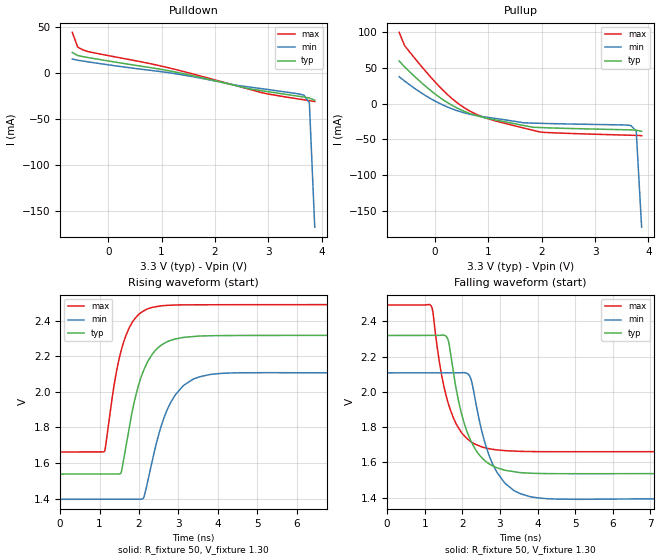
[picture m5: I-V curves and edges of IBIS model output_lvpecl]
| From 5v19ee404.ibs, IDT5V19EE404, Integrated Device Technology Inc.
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[Model]   output_lvpecl
Model_type   Output_ECL
Polarity   Non-Inverting
|   typ   min   max
C_comp   2pF   1.5pF   2.5pF
Vmeas = 1.95V
Rref = 50
Cref = 0
Vref = 1.3V
|   typ   min   max
[Voltage range]   3.3V   3.135V   3.465V
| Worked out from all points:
|   rising waveform, R_fixture 50, V_fixture 1.30: 20-80 % time 534ps typ, 606ps min, 451ps max; typ from 1.54 V to 2.32 V
|   falling waveform, R_fixture 50, V_fixture 1.30: 20-80 % time 574ps typ, 609ps min, 527ps max; typ from 2.32 V to 1.54 V
[Pulldown]
|Voltage   I (typ)   I (min)   I (max)
|Note, modeling breaks down at 250mA and above.  This is well beyond the functional   |
|operating range of the device.  Should this scenario occur, catastrophic failure and   |
|possible damage to the device and/or board is of higher concern than the I-V curve   |
|behavior.  The IBIS checker will flag currents in excess of 10A with warnings.  Lines   |
|with currents in excess of 0.35 A have been commented out.  The points still remain|
|available to the user if the user desires to use them.   |
|-3.30000e+00   3.30641e+01   2.49914e+01   4.38849e+01
|-3.19898e+00   3.16607e+01   2.38842e+01   4.20980e+01
|-3.09796e+00   3.02581e+01   2.27777e+01   4.03117e+01
|-2.99694e+00   2.88562e+01   2.16720e+01   3.85264e+01
|-2.89592e+00   2.74551e+01   2.05672e+01   3.67423e+01
|-2.79490e+00   2.60551e+01   1.94634e+01   3.49594e+01
|-2.69388e+00   2.46561e+01   1.83607e+01   3.31775e+01
|-2.59286e+00   2.32583e+01   1.72592e+01   3.13966e+01
|-2.49184e+00   2.18620e+01   1.61591e+01   2.96168e+01
|-2.39082e+00   2.04675e+01   1.50607e+01   2.78382e+01
|-2.28980e+00   1.90751e+01   1.39641e+01   2.60611e+01
|-2.18878e+00   1.76846e+01   1.28696e+01   2.42857e+01
|-2.08776e+00   1.62964e+01   1.17779e+01   2.25121e+01
|-1.98673e+00   1.49107e+01   1.06894e+01   2.07407e+01
|-1.88571e+00   1.35280e+01   9.60463e+00   1.89718e+01
|-1.78469e+00   1.21491e+01   8.52420e+00   1.72060e+01
|-1.68367e+00   1.07746e+01   7.44910e+00   1.54439e+01
|-1.58265e+00   9.40591e+00   6.38088e+00   1.36863e+01
|-1.48163e+00   8.04461e+00   5.32189e+00   1.19346e+01
|-1.38061e+00   6.69331e+00   4.27582e+00   1.01904e+01
|-1.27959e+00   5.35620e+00   3.24912e+00   8.45656e+00
|-1.17857e+00   4.04066e+00   2.25420e+00   6.73744e+00
|-1.07755e+00   2.76142e+00   1.31931e+00   5.04113e+00
|-9.76531e-01   1.55427e+00   5.24768e-01   3.38438e+00
|-8.75510e-01   5.35619e-01   9.10535e-02   1.81128e+00
|-7.74490e-01   6.46367e-02   2.16971e-02   4.96338e-01
-673.5mV  22.71mA    15.59mA    44.66mA
-572.4mV  19.44mA    14.32mA    28.67mA
-471.4mV  18.21mA    13.39mA    25.45mA
-370.4mV  17.17mA    12.49mA    23.61mA
1.044V    3.829mA    1.478mA    7.282mA
1.549V    -2.056mA   -3.223mA   -51.59uA
2.357V    -12.83mA   -12.46mA   -12.7mA
2.66V     -16.9mA    -14.93mA   -17.5mA
2.963V    -19.58mA   -17.29mA   -22.04mA
3.67V     -25.75mA   -23.67mA   -28.75mA
3.771V    -26.86mA   -32.04mA   -29.63mA
3.872V    -29.23mA   -167.3mA   -30.63mA
| 3.97347e+00   -3.47071e-02   -1.04797e+00   -3.28632e-02
| 4.07449e+00   -7.42742e-02   -2.67305e+00   -3.86876e-02
| 4.17551e+00   -7.36046e-01   -4.58869e+00   -4.80592e-02
| 4.27653e+00   -2.68947e+00   -6.62812e+00   -6.21080e-02
| 4.37755e+00   -5.16615e+00   -8.73294e+00   -3.32880e-01
| 4.47857e+00   -7.82753e+00   -1.08776e+01   -2.58593e+00
| 4.57959e+00   -1.05770e+01   -1.30488e+01   -6.00998e+00
| 4.68061e+00   -1.33771e+01   -1.52389e+01   -9.74161e+00
| 4.78163e+00   -1.62098e+01   -1.74432e+01   -1.35985e+01
| 4.88265e+00   -1.90653e+01   -1.96585e+01   -1.75220e+01
| 4.98367e+00   -2.19374e+01   -2.18826e+01   -2.14866e+01
| 5.08469e+00   -2.48223e+01   -2.41146e+01   -2.54789e+01
| 5.18571e+00   -2.77173e+01   -2.63531e+01   -2.94912e+01
| 5.28673e+00   -3.06204e+01   -2.85968e+01   -3.35185e+01
| 5.38776e+00   -3.35301e+01   -3.08448e+01   -3.75575e+01
| 5.48878e+00   -3.64456e+01   -3.30966e+01   -4.16060e+01
| 5.58980e+00   -3.93662e+01   -3.53516e+01   -4.56621e+01
| 5.69082e+00   -4.22918e+01   -3.76094e+01   -4.97246e+01
| 5.79184e+00   -4.52214e+01   -3.98697e+01   -5.37926e+01
| 5.89286e+00   -4.81542e+01   -4.21323e+01   -5.78652e+01
| 5.99388e+00   -5.10899e+01   -4.43969e+01   -6.19419e+01
| 6.09490e+00   -5.40281e+01   -4.66634e+01   -6.60221e+01
| 6.19592e+00   -5.69685e+01   -4.89314e+01   -7.01060e+01
| 6.29694e+00   -5.99109e+01   -5.12010e+01   -7.41936e+01
| 6.39796e+00   -6.28552e+01   -5.34719e+01   -7.82839e+01
| 6.49898e+00   -6.58011e+01   -5.57441e+01   -8.23765e+01
| 6.60000e+00   -6.87485e+01   -5.80174e+01   -8.64711e+01
[Pullup]
|Voltage   I (typ)   I (min)   I (max)
|Note, modeling breaks down at 250mA and above.  This is well beyond the functional   |
|operating range of the device.  Should this scenario occur, catastrophic failure and   |
|possible damage to the device and/or board is of higher concern than the I-V curve   |
|behavior.  The IBIS checker will flag currents in excess of 10A with warnings.  Lines   |
|with currents in excess of 0.35 A have been commented out.  The points still remain|
|available to the user if the user desires to use them.   |
|-3.30000e+00   3.30646e+01   2.49917e+01   4.38858e+01
|-3.19898e+00   3.16613e+01   2.38845e+01   4.20992e+01
|-3.09796e+00   3.02586e+01   2.27781e+01   4.03137e+01
|-2.99694e+00   2.88568e+01   2.16724e+01   3.85290e+01
|-2.89592e+00   2.74558e+01   2.05677e+01   3.67452e+01
|-2.79490e+00   2.60558e+01   1.94639e+01   3.49621e+01
|-2.69388e+00   2.46570e+01   1.83612e+01   3.31800e+01
|-2.59286e+00   2.32594e+01   1.72598e+01   3.13989e+01
|-2.49184e+00   2.18635e+01   1.61598e+01   2.96189e+01
|-2.39082e+00   2.04694e+01   1.50614e+01   2.78402e+01
|-2.28980e+00   1.90769e+01   1.39649e+01   2.60629e+01
|-2.18878e+00   1.76863e+01   1.28707e+01   2.42873e+01
|-2.08776e+00   1.62980e+01   1.17792e+01   2.25136e+01
|-1.98673e+00   1.49122e+01   1.06908e+01   2.07421e+01
|-1.88571e+00   1.35295e+01   9.60606e+00   1.89732e+01
|-1.78469e+00   1.21505e+01   8.52558e+00   1.72074e+01
|-1.68367e+00   1.07761e+01   7.45048e+00   1.54454e+01
|-1.58265e+00   9.40743e+00   6.38232e+00   1.36879e+01
|-1.48163e+00   8.04629e+00   5.32346e+00   1.19363e+01
|-1.38061e+00   6.69525e+00   4.27765e+00   1.01924e+01
|-1.27959e+00   5.35855e+00   3.25142e+00   8.45890e+00
|-1.17857e+00   4.04369e+00   2.25736e+00   6.74033e+00
|-1.07755e+00   2.76571e+00   1.32432e+00   5.04491e+00
|-9.76531e-01   1.56136e+00   5.34702e-01   3.38984e+00
|-8.75510e-01   5.51351e-01   1.12022e-01   1.82082e+00
|-7.74490e-01   9.94522e-02   4.65435e-02   5.21672e-01
-673.5mV  59.85mA    37.79mA    99.96mA
-572.4mV  51.65mA    31.85mA    81.49mA
-269.4mV  30.37mA    15.71mA    53.55mA
33.67mV   11.68mA    2.348mA    27.77mA
437.8mV   -6.926mA   -10.31mA   28.84uA
740.8mV   -15.86mA   -16.09mA   -13.68mA
1.044V    -21.4mA    -19.66mA   -22.19mA
1.65V     -30.33mA   -26.55mA   -33.81mA
1.953V    -33.29mA   -27.42mA   -39.29mA
3.67V     -36.6mA    -30.48mA   -44.12mA
3.771V    -37.03mA   -38.18mA   -44.33mA
3.872V    -38.65mA   -172.8mA   -44.69mA
| 3.97347e+00   -4.31075e-02   -1.05342e+00   -4.62337e-02
| 4.07449e+00   -8.15915e-02   -2.67922e+00   -5.10210e-02
| 4.17551e+00   -7.43393e-01   -4.59615e+00   -5.89005e-02
| 4.27653e+00   -2.69724e+00   -6.63718e+00   -7.12793e-02
| 4.37755e+00   -5.17451e+00   -8.74377e+00   -3.41726e-01
| 4.47857e+00   -7.83699e+00   -1.08903e+01   -2.59660e+00
| 4.57959e+00   -1.05880e+01   -1.30634e+01   -6.02150e+00
| 4.68061e+00   -1.33898e+01   -1.52556e+01   -9.75386e+00
| 4.78163e+00   -1.62244e+01   -1.74619e+01   -1.36115e+01
| 4.88265e+00   -1.90818e+01   -1.96793e+01   -1.75361e+01
| 4.98367e+00   -2.19559e+01   -2.19053e+01   -2.15021e+01
| 5.08469e+00   -2.48428e+01   -2.41385e+01   -2.54961e+01
| 5.18571e+00   -2.77398e+01   -2.63776e+01   -2.95102e+01
| 5.28673e+00   -3.06450e+01   -2.86217e+01   -3.35395e+01
| 5.38776e+00   -3.35569e+01   -3.08701e+01   -3.75806e+01
| 5.48878e+00   -3.64744e+01   -3.31221e+01   -4.16311e+01
| 5.58980e+00   -3.93968e+01   -3.53773e+01   -4.56893e+01
| 5.69082e+00   -4.23232e+01   -3.76353e+01   -4.97540e+01
| 5.79184e+00   -4.52533e+01   -3.98959e+01   -5.38241e+01
| 5.89286e+00   -4.81864e+01   -4.21586e+01   -5.78989e+01
| 5.99388e+00   -5.11224e+01   -4.44234e+01   -6.19778e+01
| 6.09490e+00   -5.40609e+01   -4.66900e+01   -6.60602e+01
| 6.19592e+00   -5.70015e+01   -4.89582e+01   -7.01457e+01
| 6.29694e+00   -5.99442e+01   -5.12279e+01   -7.42340e+01
| 6.39796e+00   -6.28887e+01   -5.34990e+01   -7.83248e+01
| 6.49898e+00   -6.58349e+01   -5.57713e+01   -8.24178e+01
| 6.60000e+00   -6.87825e+01   -5.80448e+01   -8.65128e+01
[Ramp]
|   typ   min   max
dV/dt_r   0.467/0.533n   0.426/0.609n   0.497/0.451n
dV/dt_f   0.471/0.575n   0.43/0.619n   0.5/0.528n
R_load =   50.0000
[Rising Waveform]
R_fixture = 50
V_fixture = 1.30   | VCC_typ - 2V
V_fixture_max = 1.465   | VCC_max - 2V
V_fixture_min = 1.135   | VCC_min - 2V
C_fixture = 0.0p
| Time   typ   min   max
0s        1.538V     1.397V     1.663V
1.127ns   1.538V     1.397V     1.667V
1.371ns   1.538V     1.397V     2.041V
1.541ns   1.544V     1.397V     2.227V
1.902ns   1.964V     1.397V     2.413V
2.105ns   2.114V     1.401V     2.453V
2.213ns   2.167V     1.489V     2.467V
2.718ns   2.282V     1.901V     2.486V
3.383ns   2.311V     2.073V     2.489V
10ns      2.318V     2.107V     2.491V
[Falling Waveform]
R_fixture = 50
V_fixture = 1.30   | VCC_typ - 2V
V_fixture_max = 1.465   | VCC_max - 2V
V_fixture_min = 1.135   | VCC_min - 2V
C_fixture = 0.0p
| Time   typ   min   max
0s        2.319V     2.108V     2.492V
1.173ns   2.319V     2.108V     2.487V
1.412ns   2.32V      2.108V     2.143V
1.582ns   2.312V     2.108V     1.97V
1.928ns   1.922V     2.108V     1.786V
2.199ns   1.736V     2.089V     1.722V
2.5ns     1.631V     1.794V     1.69V
2.93ns    1.569V     1.542V     1.671V
3.75ns    1.54V      1.409V     1.662V
10ns      1.537V     1.395V     1.662V
